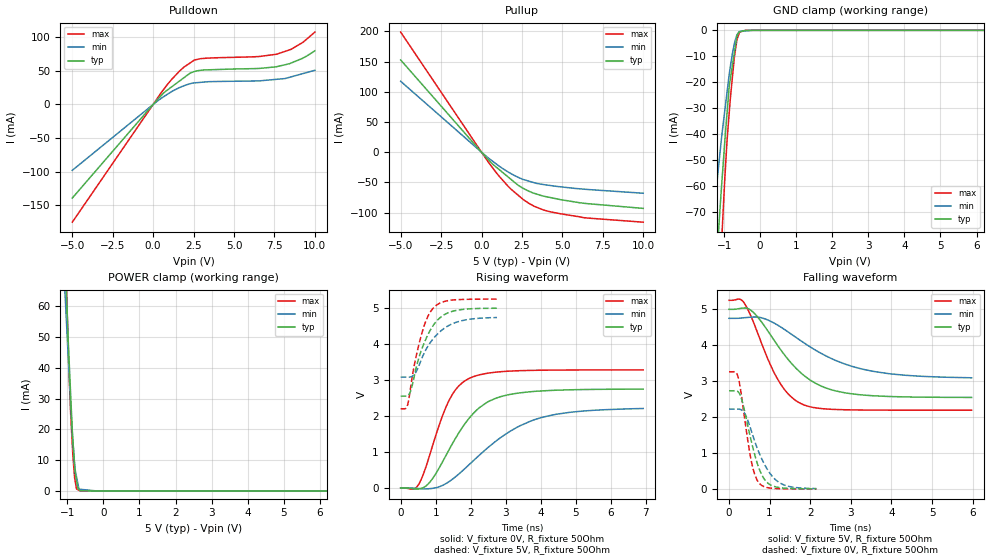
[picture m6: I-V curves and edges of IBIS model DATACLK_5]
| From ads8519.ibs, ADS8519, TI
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|   dataclk_5 Model
[Model]   DATACLK_5
Model_type   I/O
Polarity   Non-Inverting
Enable   Active-Low
Vinl = 0.6
Vinh = 2.5
Vmeas = 2.5
Vref = 2.5
Cref = 15pF
Rref = 50
|   typ   min   max
|   (nom PVT)   (Fast PVT)   (slow PVT)
| C_comp by Frequency method (F=29Mhz)
|Average
|C_comp   8.842e-12   7.883e-12   9.912e-12
|ON state : BUFFER OUTPUT TURNED HIGH
|C_comp   1.005e-11   9.006e-12   1.136e-11
|OFF state: BUFFER IN HIGH IMPEDANCE
|C_comp   7.635e-12   6.760e-12   8.463e-12
| C_comp by LC Tank method (L=1nH)
| Resonant frequency (Hz) 1.88e9   1.96e9   1.8e9
|Average
C_comp   7.177e-12   6.570e-12   8.914e-12
| Where nom  PVT is Nominal Process,  5V,  32C
|   Fast PVT is Strong Process,   5.25V,  -40C
|   Slow PVT is Weak Process,   4.75V,  92C
[Model Spec]
Vinl   0.6   0.6   0.6
Vinh   2.5   2.375   2.625
[Voltage Range]   5   4.75   5.25
|Ambient Temperature   25   85   -40
|Junction Temperature
[Temperature Range]   32   92   -40
[Pullup Reference]   5   4.75   5.25
[Pulldown Reference]   0   0   0
[Power Clamp Reference]   5   4.75   5.25
[GND Clamp Reference]   0   0   0
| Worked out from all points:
|   slope of the pulldown table from 0 to 0.75 V, typ, clamps not added: 39.4 ohm
|   slope of the pullup table from 0 to 0.75 V, typ, clamps not added: 35.3 ohm
|   GND clamp passes 1 mA (typ) near -0.60 V on its own axis
|   POWER clamp passes 1 mA (typ) near -0.71 V on its own axis
|   falling waveform, V_fixture 5V, R_fixture 50Ohm: 20-80 % time 1.1ns typ, 1.6ns min, 740ps max; typ from 5 V to 2.55 V
|   rising waveform, V_fixture 0V, R_fixture 50Ohm: 20-80 % time 1.11ns typ, 1.77ns min, 747ps max; typ from 0 V to 2.75 V
|   rising waveform, V_fixture 5V, R_fixture 50Ohm: 20-80 % time 548ps typ, 674ps min, 433ps max; typ from 2.55 V to 4.99 V
|   falling waveform, V_fixture 0V, R_fixture 50Ohm: 20-80 % time 368ps typ, 494ps min, 269ps max; typ from 2.74 V to 0.013 V
[Pulldown]
|   Voltage   I(typ)   I(min)   I(max)
-5V       -139.1mA   -97.9mA    -174.9mA
255mV     6.981mA    4.834mA    8.994mA
700mV     18.15mA    12.28mA    23.9mA
1.145V    26.11mA    19.09mA    37.2mA
1.906V    39.76mA    27.76mA    55.49mA
2.551V    48.92mA    32.07mA    66mA
2.94V     50.78mA    32.86mA    68.06mA
6.557V    53.53mA    35.02mA    71.22mA
7.644V    56.16mA    37.38mA    74.68mA
8.537V    61.59mA    41.01mA    81.97mA
9.271V    69mA       45.91mA    92.47mA
10V       79.7mA     50.77mA    107.5mA
[GND Clamp]
|   Voltage   I(typ)   I(min)   I(max)
-5V       -998.9mA   -733.2mA   -1.367A
-1.31V    -110.1mA   -73.92mA   -156.2mA
-1.165V   -79.75mA   -54.17mA   -110.8mA
-1.088V   -63.44mA   -43.57mA   -87.42mA
-1.055V   -57.12mA   -39.49mA   -77.7mA
-924mV    -32.83mA   -24.46mA   -43.7mA
-855mV    -21.22mA   -16.57mA   -31.23mA
-824.3mV  -18.45mA   -13.73mA   -25.81mA
-714mV    -8.521mA   -5.051mA   -10.17mA
-640mV    -1.854mA   -1.682mA   -3.4mA
-574.7mV  -594.2uA   -427.5uA   -851.3uA
10V       0A         0A         0A
[Pullup]
|   Voltage   I(typ)   I(min)   I(max)
-5V       152.6mA    117.3mA    198.7mA
404.2mV   -11.9mA    -9.156mA   -15.79mA
1.066V    -28.22mA   -22.63mA   -39mA
1.596V    -39.97mA   -31.97mA   -55.04mA
2.27V     -54.91mA   -41.66mA   -71.37mA
2.599V    -60.1mA    -45.33mA   -78.81mA
3.271V    -68.18mA   -50.65mA   -89.69mA
3.838V    -72.81mA   -53.62mA   -95.66mA
4.956V    -78.92mA   -57.54mA   -102.3mA
6.557V    -85.21mA   -61.74mA   -109mA
10V       -93.07mA   -67.96mA   -115.9mA
[POWER Clamp]
|   Voltage   I(typ)   I(min)   I(max)
-5V       1.402A     1.206A     1.7A
-1.076V   80.8mA     66.9mA     88.95mA
-1.013V   60.65mA    52.18mA    61.25mA
-955.5mV  43.37mA    38.69mA    39.07mA
-908.3mV  31.14mA    27.75mA    24.94mA
-855mV    17.79mA    17.3mA     13.26mA
-798mV    8.206mA    8.321mA    4.151mA
-785mV    6.02mA     6.928mA    3.276mA
-745.5mV  3.384mA    4.556mA    616.5uA
-705mV    681.2uA    2.124mA    380.6uA
-640.5mV  71.81uA    531.5uA    4.903uA
10V       0A         0A         0A
[Ramp]
R_load = 50
|   typ   min   max
dV/dt_r   1.6487/1.11438e-09   1.34034/1.8074e-09   1.96688/7.4717e-10
dV/dt_f   1.46995/1.10385e-09   1.00307/1.64288e-09   1.83103/7.39576e-10
[Falling Waveform]
V_fixture = 5V
V_fixture_min = 4.75V
V_fixture_max = 5.25V
R_fixture = 50Ohm
|   Time   V(typ)   V(min)   V(max)
0s        5V         4.75V      5.25V
250ps     5.02V      4.753V     5.285V
375ps     5.037V     4.767V     5.174V
675ps     4.826V     4.787V     4.43V
1.2ns     3.993V     4.56V      3.055V
1.5ns     3.548V     4.337V     2.601V
1.8ns     3.205V     4.103V     2.366V
2.4ns     2.81V      3.699V     2.232V
3.35ns    2.615V     3.323V     2.203V
5.975ns   2.553V     3.098V     2.198V
[Rising Waveform]
V_fixture = 0V
V_fixture_min = 0V
V_fixture_max = 0V
R_fixture = 50Ohm
|   Time   V(typ)   V(min)   V(max)
0s        3.744nV    4.393nV    3.296nV
500ps     -29.92mV   -16.69mV   74.91mV
825ps     150.6mV    -21.96mV   900.1mV
1.35ns    1.004V     153.9mV    2.367V
1.625ns   1.474V     356.5mV    2.796V
1.95ns    1.93V      642.2mV    3.039V
2.7ns     2.485V     1.285V     3.215V
3.875ns   2.686V     1.912V     3.268V
5ns       2.73V      2.118V     3.277V
6.925ns   2.745V     2.207V     3.278V
[Rising Waveform]
V_fixture = 5V
V_fixture_min = 4.75V
V_fixture_max = 5.25V
R_fixture = 50Ohm
|   Time   V(typ)   V(min)   V(max)
0s        2.55V      3.078V     2.198V
200ps     2.562V     3.078V     2.309V
300ps     2.738V     3.088V     2.896V
400ps     3.156V     3.165V     3.462V
575ps     3.781V     3.527V     4.189V
750ps     4.2V       3.892V     4.707V
925ps     4.508V     4.14V      4.99V
1.175ns   4.769V     4.384V     5.157V
1.5ns     4.913V     4.571V     5.223V
2.75ns    4.993V     4.735V     5.248V
[Falling Waveform]
V_fixture = 0V
V_fixture_min = 0V
V_fixture_max = 0V
R_fixture = 50Ohm
|   Time   V(typ)   V(min)   V(max)
0s        2.738V     2.23V      3.265V
150ps     2.739V     2.23V      3.261V
225ps     2.71V      2.229V     3.113V
375ps     2.215V     2.128V     2.045V
525ps     1.45V      1.71V      923.5mV
625ps     995.8mV    1.363V     443.4mV
725ps     624.1mV    1.057V     195.5mV
925ps     206.7mV    589.4mV    53.63mV
1.225ns   51.85mV    198.1mV    17.98mV
2.15ns    12.63mV    21.66mV    4.935mV
